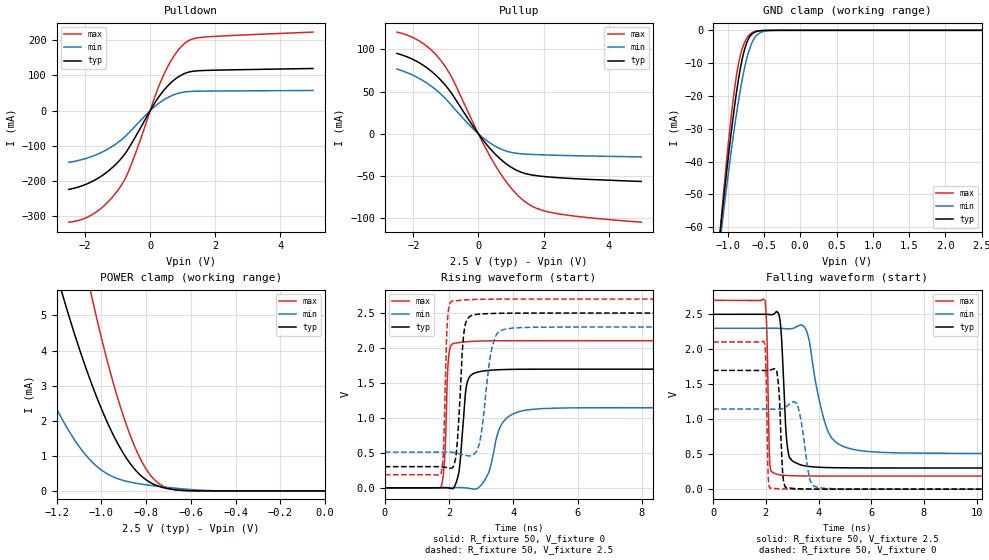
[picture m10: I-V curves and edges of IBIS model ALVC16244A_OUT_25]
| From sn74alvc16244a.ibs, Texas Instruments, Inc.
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[Model]   ALVC16244A_OUT_25
Model_type  3-state
Enable   Active-Low
Vref =   0
Rref =   500
Cref =   30p
Vmeas =   1.25
| variable   typ   min   max
C_comp   2.49pF   2.17pF   2.60pF
| C_pullup   3.53pF   3.04pF   4.42pF
| C_pulldown   4.78pF   2.99pF   6.82pF
| C_tri-state   2.49pF   2.17pF   2.60pF
[Temperature Range]   40   100   -40
| Ambient temperature   25   85   -40
[Voltage range]   2.5   2.3   2.7
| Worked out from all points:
|   slope of the pulldown table from 0 to 0.375 V, typ, clamps not added: 7.11 ohm
|   slope of the pullup table from 0 to 0.375 V, typ, clamps not added: 20.7 ohm
|   GND clamp passes 1 mA (typ) near -0.66 V on its own axis
|   POWER clamp passes 1 mA (typ) near -0.89 V on its own axis
|   rising waveform, R_fixture 50, V_fixture 0: 20-80 % time 175ps typ, 404ps min, 96ps max; typ from 0 V to 1.7 V
|   falling waveform, R_fixture 50, V_fixture 2.5: 20-80 % time 171ps typ, 592ps min, 79.6ps max; typ from 2.5 V to 0.303 V
|   rising waveform, R_fixture 50, V_fixture 2.5: 20-80 % time 161ps typ, 278ps min, 90.8ps max; typ from 0.303 V to 2.5 V
|   falling waveform, R_fixture 50, V_fixture 0: 20-80 % time 116ps typ, 258ps min, 65.7ps max; typ from 1.7 V to 0 V
[GND Clamp]
| ALVC16244A_OUT_25
|   Voltage   I(typ)   I(min)   I(max)
-2.5V     -421.6mA   -385.2mA   -473mA
-1.1V     -61.03mA   -63.82mA   -60.43mA
-1.08V    -56.79mA   -60.03mA   -55.48mA
-1.06V    -52.61mA   -56.29mA   -50.61mA
-950mV    -31.09mA   -36.84mA   -26.11mA
-870mV    -17.8mA    -24.35mA   -12.7mA
-820mV    -11.13mA   -17.57mA   -7.281mA
-765mV    -5.73mA    -11.32mA   -3.638mA
-655mV    -955.9uA   -3.345mA   -636.6uA
-560mV    -152.2uA   -821.8uA   -112.4uA
-425mV    -10.46uA   -85.14uA   -10.28uA
2.5V      2.145nA    60.35nA    10.72nA
[POWER Clamp]
| ALVC16244A_OUT_25
|   Voltage   I(typ)   I(min)   I(max)
-2.5V     56.58mA    36.27mA    85.37mA
-1.405V   11.53mA    5.461mA    19.19mA
-1.28V    8.118mA    3.43mA     13.78mA
-1.175V   5.632mA    2.045mA    9.78mA
-1.045V   3.081mA    848uA      5.599mA
-955mV    1.705mA    424uA      3.269mA
-885mV    906.7uA    271uA      1.829mA
-815mV    391.2uA    188.8uA    788.2uA
-750mV    147.6uA    134.7uA    246.1uA
-690mV    50.51uA    92.43uA    57.6uA
-615mV    8.309uA    47.17uA    6.732uA
-31.15fV  2.145nA    59.67nA    10.48nA
[Pulldown]
| ALVC16244A_OUT_25
|   Voltage   I(typ)   I(min)   I(max)
-2.5V     -223.3mA   -146.6mA   -316.5mA
-2.06V    -212.2mA   -137.9mA   -307.4mA
-1.655V   -194.7mA   -125mA     -287.5mA
-1.26V    -169.4mA   -106.8mA   -255.7mA
-895mV    -136.5mA   -83.49mA   -213.1mA
-540mV    -88.14mA   -51.89mA   -143.3mA
145mV     22.52mA    12.19mA    39.65mA
395mV     55.03mA    29.41mA    97.31mA
740mV     87.57mA    45.62mA    156.4mA
1.085V    106.6mA    53.52mA    192.9mA
1.685V    114.3mA    55.59mA    209.1mA
5V        119.8mA    57.44mA    223.2mA
[Pullup]
| ALVC16244A_OUT_25
|   Voltage   I(typ)   I(min)   I(max)
-2.5V     95.2mA     76.65mA    120.5mA
-1.735V   82.23mA    63.78mA    108mA
-1.41V    72.97mA    55.35mA    97.9mA
-1.12V    62.15mA    45.9mA     85.18mA
-780mV    45.42mA    31.75mA    64.07mA
-165mV    9.08mA     6.027mA    13.33mA
285mV     -14.15mA   -8.875mA   -21.52mA
865mV     -35.79mA   -20.44mA   -57.31mA
1.41V     -46.63mA   -23.86mA   -79.68mA
1.81V     -49.62mA   -24.62mA   -88.48mA
2.38V     -51.69mA   -25.33mA   -94.16mA
5V        -56.32mA   -27.28mA   -104.6mA
[Ramp]
| ALVC16244A_OUT_25
| variable   typ   min   max
dV/dt_r   1.03/1.83E-10   0.70/4.17E-10   1.27/1.03E-10
dV/dt_f   1.34/1.91E-10   1.10/6.05E-10   1.52/8.27E-11
R_load = 50
[Rising Waveform]
| ALVC16244A_OUT_25
R_fixture =   50
C_fixture =   0
L_fixture =   0
V_fixture =   0
V_fixture_min = 0
V_fixture_max = 0
|   Time   V(typ)   V(min)   V(max)
0s        270.5pV    431.1pV    174.2pV
1.75ns    1.391mV    -145.7uV   11.91mV
1.87ns    3.776mV    -117.6uV   480.9mV
2.005ns   -3.85mV    565.7uV    1.942V
2.305ns   216.6mV    4.744mV    2.077V
2.525ns   1.412V     -1.13mV    2.089V
3.145ns   1.675V     137mV      2.102V
3.765ns   1.692V     984.1mV    2.104V
4.905ns   1.697V     1.134V     2.105V
50ns      1.697V     1.146V     2.105V
[Falling Waveform]
| ALVC16244A_OUT_25
R_fixture =   50
C_fixture =   0
L_fixture =   0
V_fixture =   2.5
V_fixture_min = 2.3
V_fixture_max = 2.7
|   Time   V(typ)   V(min)   V(max)
0s        2.5V       2.3V       2.7V
1.975ns   2.499V     2.3V       2.696V
2.035ns   2.499V     2.3V       2.309V
2.155ns   2.496V     2.3V       356.6mV
2.545ns   2.392V     2.299V     203.8mV
2.865ns   497.9mV    2.292V     194.1mV
3.655ns   324.2mV    2.111V     188.3mV
4.415ns   308.2mV    782.4mV    187.3mV
5.865ns   303.4mV    538.9mV    187mV
50ns      302.8mV    510.5mV    187mV
[Rising Waveform]
| ALVC16244A_OUT_25
R_fixture =   50
C_fixture =   0
L_fixture =   0
V_fixture =   2.5
V_fixture_min = 2.3
V_fixture_max = 2.7
|   Time   V(typ)   V(min)   V(max)
0s        302.8mV    510.5mV    187mV
1.75ns    301.7mV    511.7mV    204.9mV
1.82ns    298.9mV    512.1mV    482mV
1.95ns    287.4mV    512.5mV    2.392V
2.135ns   309.8mV    507.1mV    2.674V
2.485ns   2.292V     466.5mV    2.687V
2.9ns     2.483V     573.2mV    2.696V
3.39ns    2.495V     2.094V     2.699V
4.025ns   2.499V     2.288V     2.7V
50ns      2.5V       2.3V       2.7V
[Falling Waveform]
| ALVC16244A_OUT_25
R_fixture =   50
C_fixture =   0
L_fixture =   0
V_fixture =   0
V_fixture_min = 0
V_fixture_max = 0
|   Time   V(typ)   V(min)   V(max)
0s        1.697V     1.146V     2.105V
1.925ns   1.697V     1.145V     2.108V
1.99ns    1.697V     1.145V     1.897V
2.09ns    1.699V     1.144V     201.8mV
2.17ns    1.704V     1.143V     10.67mV
2.435ns   1.64V      1.142V     6.527mV
2.645ns   210.2mV    1.152V     3.447mV
2.805ns   17.05mV    1.189V     2.236mV
4.285ns   502.5uV    10.02mV    71.14uV
50ns      3.214nV    -4.458nV   -327.9pV
